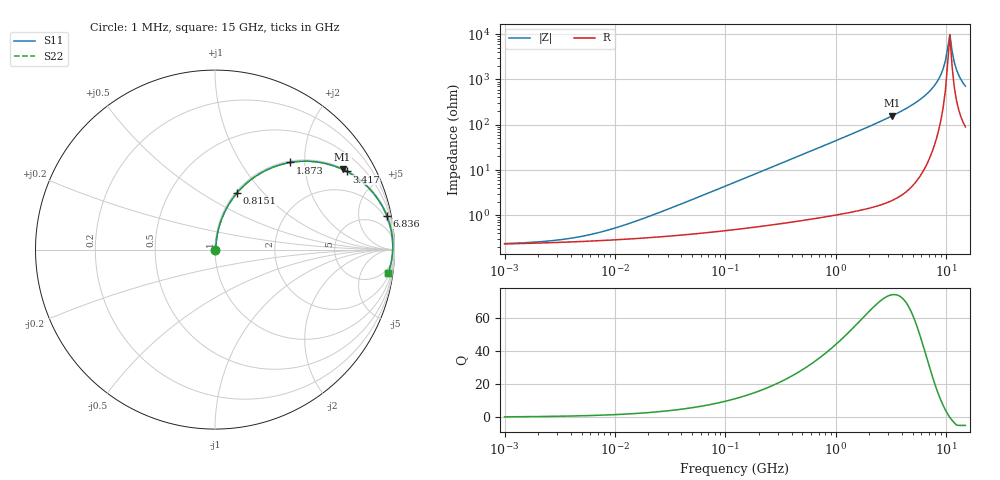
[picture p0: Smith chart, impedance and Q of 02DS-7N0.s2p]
# MHz S MA R 50
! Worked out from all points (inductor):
!   209 points, 1 MHz to 15 GHz, reference 50 ohm
!   read as one part in series: L = 7 nH near 23.19 MHz
!   highest Q = 73.6 at 3.262 GHz (marker M1), where L = 7.7 nH
!   self-resonance near 10.36 GHz
!   S11 on the Smith chart (normalised r, x): 1 MHz: 1.00, +0.00; 815.1 MHz: 1.02, +0.72; 1.873 GHz: 1.03, +1.70; 3.417 GHz: 1.05, +3.34; 6.836 GHz: 1, +10; 15 GHz: 3, -14
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1  0.002385 10.6  0.9977 -0.0  0.9977 -0.0  0.002385 10.6
5.04322  0.003455 39.7  0.9973 -0.1  0.9973 -0.1  0.003455 39.7
10.5668  0.005469 57.7  0.9971 -0.3  0.9971 -0.3  0.005469 57.7
25.434  0.01164 72.6  0.9966 -0.6  0.9966 -0.6  0.01164 72.6
128.269  0.05627 81.8  0.9935 -3.2  0.9935 -3.2  0.05627 81.8
617.665  0.2611 73.1  0.9574 -15.1  0.9574 -15.1  0.2611 73.1
815.112  0.3365 68.9  0.933 -19.7  0.933 -19.7  0.3365 68.9
1873.31  0.6423 49.1  0.7561 -40.0  0.7561 -40.0  0.6423 49.1
3115.02  0.8259 33.5  0.5527 -55.7  0.5527 -55.7  0.8259 33.5
3262.41  0.8397 32.1  0.5318 -57.1  0.5318 -57.1  0.8397 32.1
3416.77  0.8528 30.7  0.5107 -58.5  0.5107 -58.5  0.8528 30.7
5179.79  0.9425 18.6  0.3187 -70.4  0.3187 -70.4  0.9425 18.6
6835.59  0.9751 11.2  0.1947 -77.1  0.1947 -77.1  0.9751 11.2
8224.05  0.9866 6.6  0.1151 -80.0  0.1151 -80.0  0.9866 6.6
9447.52  0.9903 3.2  0.05691 -78.6  0.05691 -78.6  0.9903 3.2
9894.53  0.9907 2.1  0.03799 -74.7  0.03799 -74.7  0.9907 2.1
10853  0.99 -0.1  0.01008 8.5  0.01008 8.5  0.99 -0.1
11366.5  0.9891 -1.2  0.02332 61.4  0.02332 61.4  0.9891 -1.2
11904.3  0.9876 -2.3  0.04153 71.5  0.04153 71.5  0.9876 -2.3
12467.6  0.9857 -3.4  0.06037 74.6  0.06037 74.6  0.9857 -3.4
13675.3  0.9806 -5.6  0.09852 75.8  0.09852 75.8  0.9806 -5.6
15000  0.9734 -7.8  0.137 74.9  0.137 74.9  0.9734 -7.8
